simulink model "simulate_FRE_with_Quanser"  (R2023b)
settings: Solver=daessc  StartTime=0.0  StopTime=sim_stop_time  RelTol=1e-3
undefined symbols (not defined in the file or in its folder): dphi0, dtheta0, phi0, theta0
libraries: pendulumLib x1

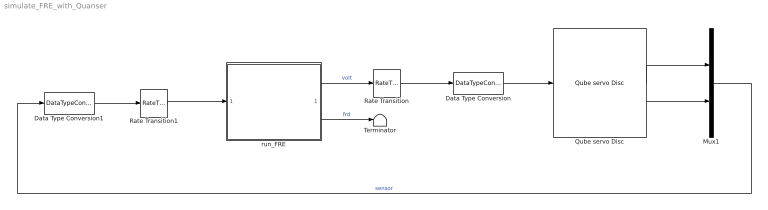
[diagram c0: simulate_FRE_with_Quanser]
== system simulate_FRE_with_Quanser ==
  Data Type Conversion : DataTypeConversion  OutDataTypeStr=double
  Data Type Conversion1 : DataTypeConversion  OutDataTypeStr=single
  Mux1 : Mux  Inputs=2
  Qube servo Disc : pendulumLib/Qube servo Disc  a0=[theta0, phi0]  w0=[dtheta0, dphi0]  R_m=R_m  L_m=L_m  mu_m=mu_m  K_b=K_b  n=n  rod_mass=m_r  rod_length=L_r  rod_rad=rod_rad  p_mass=m_p  p_length=L_p  p_rad=p_rad  D_r=D_r  D_p=D_p
  Rate Transition : RateTransition
  Rate Transition1 : RateTransition  OutPortSampleTime=FRE_time_step
  Terminator : Terminator
  run_FRE : ModelReference  ModelNameDialog=run_FRE.slx  SimulationMode=Normal  ModelReferenceVersion=1.29
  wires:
  Qube servo Disc/2 -> Mux1/2
  Qube servo Disc/1 -> Mux1/1
  run_FRE/1 -> Rate Transition/1  "volt"
  run_FRE/2 -> Terminator/1  "frd"
  Rate Transition/1 -> Data Type Conversion/1
  Data Type Conversion/1 -> Qube servo Disc/1
  Rate Transition1/1 -> run_FRE/1
  Mux1/1 -> Data Type Conversion1/1  "sensor"
  Data Type Conversion1/1 -> Rate Transition1/1
